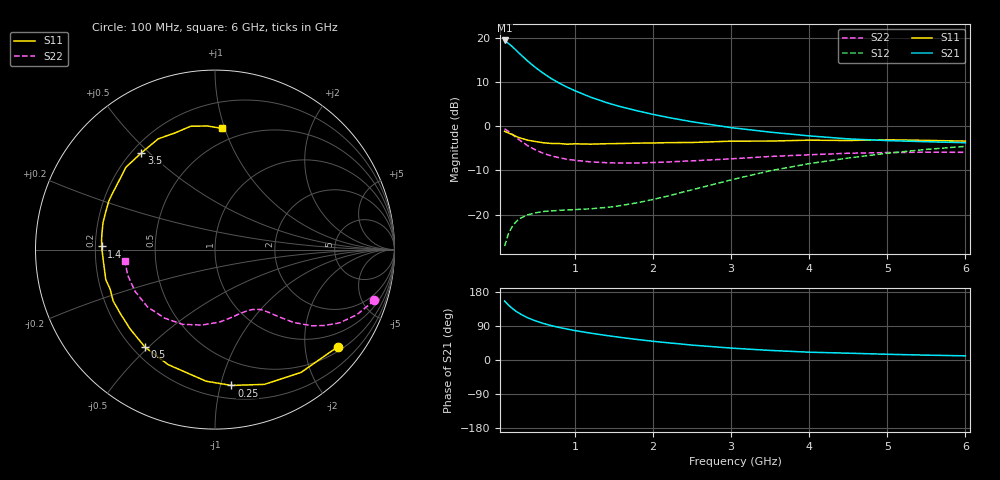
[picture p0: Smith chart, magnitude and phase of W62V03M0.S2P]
! SIEMENS Small Signal Semiconductors
! BFR193W
! Si NPN RF Bipolar Junction Transistor in SOT323
! VCE = 2 V  IC = 3 mA
! Common Emitter S-Parameters:  September  1992
# GHz  S  MA  R  50
!  f  S11  S21  S12  S22
! GHz  MAG  ANG  MAG  ANG  MAG  ANG  MAG  ANG
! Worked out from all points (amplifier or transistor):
!   28 points, 100 MHz to 6 GHz, reference 50 ohm
!   highest |S21| = 19.4 dB at 100 MHz (marker M1)
!   |S21| within 3 dB of that: start of sweep to 293.6 MHz
!   unconditionally stable (mu >= 1): 1.358 GHz to 2.614 GHz
!   at 300 MHz: K = 0.26, MSG = 18.5 dB, |S12| = -20.8 dB
!   at 1.5 GHz: K = 1.05, MAG = 10.1 dB, |S12| = -18.2 dB
!   at 6 GHz: K = 0.95, MSG = 0.4 dB, |S12| = -4.6 dB
!   S11 on the Smith chart (normalised r, x): 100 MHz: 0.61, -2.77; 250 MHz: 0.30, -1.08; 500 MHz: 0.25, -0.49; 1.4 GHz: 0.23, +0.01; 3.5 GHz: 0.24, +0.47; 6 GHz: 0.39, +0.98
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0.1  0.8731 -38.2  9.279 155.6  0.044 69.7  0.9319 -17.7
0.15  0.8355 -55.0  8.586 144.9  0.0613 61.5  0.8694 -24.7
0.2  0.7997 -69.9  7.872 135.7  0.0738 54.7  0.8046 -30.5
0.25  0.7623 -83.1  7.151 128.1  0.084 49.0  0.7396 -34.9
0.3  0.7348 -93.9  6.487 121.6  0.0909 44.7  0.6864 -38.2
0.4  0.6919 -112.2  5.383 110.9  0.0998 38.9  0.5975 -42.8
0.5  0.6686 -125.7  4.555 102.9  0.105 35.5  0.5353 -45.5
0.6  0.6475 -136.8  3.931 96.3  0.1084 33.5  0.4905 -47.8
0.7  0.6366 -145.6  3.43 90.6  0.1102 32.8  0.4605 -49.4
0.8  0.6356 -153.2  3.059 85.8  0.1116 32.8  0.4385 -51.1
0.9  0.6244 -159.3  2.752 81.6  0.1128 33.5  0.4223 -52.4
1  0.631 -164.6  2.511 77.7  0.1139 34.6  0.4111 -54.1
1.2  0.6253 -173.7  2.124 70.9  0.1163 37.8  0.3941 -57.9
1.4  0.6319 178.4  1.848 64.8  0.1205 41.9  0.3861 -61.7
1.8  0.6418 166.4  1.487 54.1  0.1361 51.4  0.3832 -70.6
2.2  0.6505 155.4  1.249 45.3  0.163 58.9  0.3932 -79.9
2.5  0.6527 148.3  1.119 39.3  0.1904 62.4  0.4048 -87.1
3  0.676 137.2  0.961 31.4  0.2469 64.3  0.4267 -99.8
3.5  0.6772 127.3  0.855 25.3  0.3128 62.2  0.4537 -113.4
4.5  0.6873 108.8  0.717 18.0  0.4357 52.7  0.4934 -139.7
5.5  0.6896 93.4  0.666 12.8  0.5455 41.1  0.5071 -163.8
6  0.6764 86.8  0.649 11.0  0.5905 34.8  0.5054 -173.0
